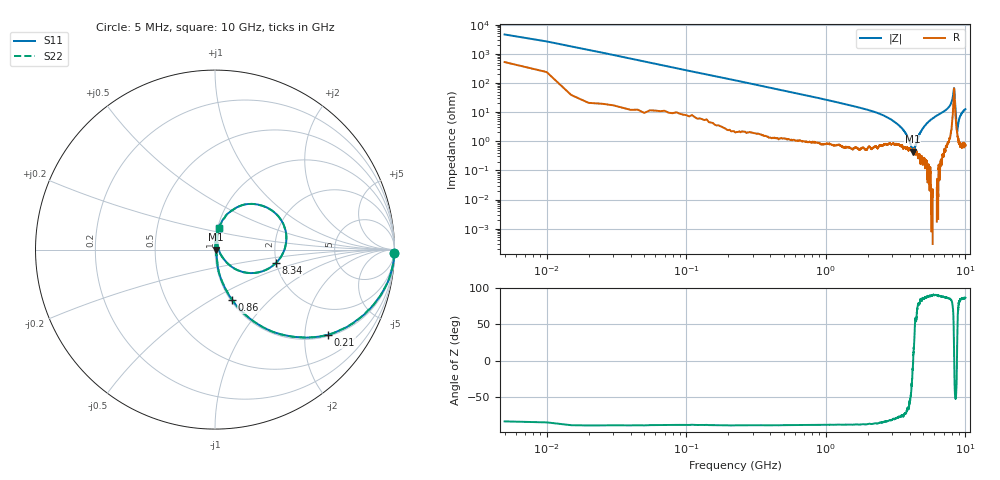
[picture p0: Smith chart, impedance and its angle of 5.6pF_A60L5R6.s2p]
! Amotech Co.,Ltd.
! http://www.amotech.co.kr/
! Part Number: A60L5R6
! These Parameters are Measured in Series Mode Connection
! Operation Temp=25[degC], DC Bias Voltage=0[V]
! Freq. Start=5[MHz] Stop=10[GHz], 2000[Steps]
! Date: Monday, July 14, 2020, 09:52:42
# GHZ S RI R 50.000000
!Freq.(Hz) S11(Real) S11(Imag) S21(Real) S21(Imag) S12(Real) S12(Imag) S22(Real) S22(Imag)
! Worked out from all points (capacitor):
!   2000 points, 5 MHz to 10 GHz, reference 50 ohm
!   read as one part in series: C = 5.85 pF near 55 MHz
!   lowest |Z| = 440 mohm at 4.195 GHz (marker M1)
!   series resonance near 4.224 GHz, so ESL is about 240 pH
!   S11 on the Smith chart (normalised r, x): 5 MHz: 11, -91; 210 MHz: 1.04, -2.62; 860 MHz: 1.02, -0.62; 8.34 GHz: 1.98, -0.34; 10 GHz: 1.01, +0.25
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0.005  0.9971 -0.0215  0.00292 0.0215  0.00292 0.0215  0.9971 -0.0215
0.085  0.9039 -0.2797  0.0961 0.2797  0.0961 0.2797  0.9039 -0.2797
0.21  0.6292 -0.4748  0.3708 0.4748  0.3708 0.4748  0.6292 -0.4748
0.465  0.2623 -0.4295  0.7377 0.4295  0.7377 0.4295  0.2623 -0.4295
0.86  0.0957 -0.28  0.9043 0.28  0.9043 0.28  0.0957 -0.28
1.675  0.0272 -0.1439  0.9728 0.1439  0.9728 0.1439  0.0272 -0.1439
3.34  0.00892 -0.0332  0.9911 0.0332  0.9911 0.0332  0.00892 -0.0332
3.805  0.00606 -0.0147  0.9939 0.0147  0.9939 0.0147  0.00606 -0.0147
4.195  0.00428 -0.00097  0.9957 0.00097  0.9957 0.00097  0.00428 -0.00097
4.7  0.00378 0.0175  0.9962 -0.0175  0.9962 -0.0175  0.00378 0.0175
5.005  0.00294 0.029  0.9971 -0.029  0.9971 -0.029  0.00294 0.029
5.645  0.00385 0.0544  0.9961 -0.0544  0.9961 -0.0544  0.00385 0.0544
6.67  0.0104 0.0901  0.9896 -0.0901  0.9896 -0.0901  0.0104 0.0901
7.69  0.0357 0.1497  0.9643 -0.1497  0.9643 -0.1497  0.0357 0.1497
8.165  0.1982 0.2546  0.8018 -0.2546  0.8018 -0.2546  0.1982 0.2546
8.27  0.3838 0.1352  0.6162 -0.1352  0.6162 -0.1352  0.3838 0.1352
8.335  0.3487 -0.0653  0.6513 0.0653  0.6513 0.0653  0.3487 -0.0653
8.34  0.338 -0.0764  0.662 0.0764  0.662 0.0764  0.338 -0.0764
8.49  0.0835 -0.0884  0.9165 0.0884  0.9165 0.0884  0.0835 -0.0884
8.72  0.0201 0.0049  0.9799 -0.0049  0.9799 -0.0049  0.0201 0.0049
9.155  0.0111 0.0681  0.9889 -0.0681  0.9889 -0.0681  0.0111 0.0681
10  0.0227 0.123  0.9773 -0.123  0.9773 -0.123  0.0227 0.123
